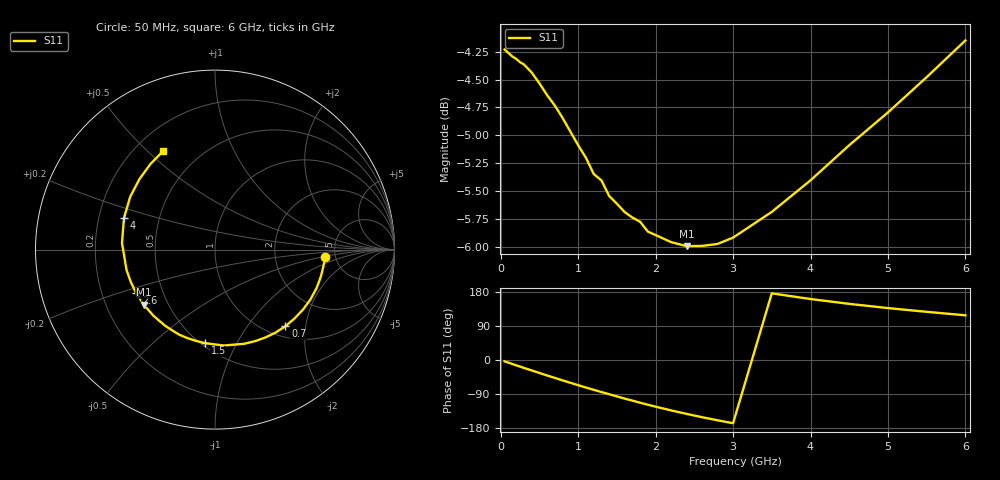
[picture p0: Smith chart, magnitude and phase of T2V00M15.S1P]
! SIEMENS Discrete & RF Semiconductors
! BAS70-04W
! Si Schottky Diode in SOT323
! IF = 0.15 mA
! S-Parameters:  November  1997
# GHz  S  MA  R  50
!  f  S11
! GHz  MAG  ANG
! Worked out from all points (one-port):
!   34 points, 50 MHz to 6 GHz, reference 50 ohm
!   lowest |S11| = -6.0 dB at 2.4 GHz (marker M1), VSWR 3.01, Z = 18.3 - j15 ohm
!   |S11| at or under -10 dB: nowhere
!   S11 on the Smith chart (normalised r, x): 50 MHz: 4.12, -0.51; 700 MHz: 1.20, -1.55; 1.5 GHz: 0.52, -0.75; 2.6 GHz: 0.35, -0.23; 4 GHz: 0.31, +0.15; 6 GHz: 0.31, +0.56
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0.05  0.6144 -3.6
0.15  0.61 -10.6
0.2  0.6085 -14.2
0.25  0.6064 -17.4
0.4  0.5999 -27.6
0.5  0.5933 -34.3
0.6  0.586 -41.0
0.7  0.5797 -47.4
0.8  0.5724 -53.9
0.9  0.5644 -60.2
1  0.5566 -66.5
1.1  0.5494 -72.7
1.3  0.5367 -84.6
1.5  0.5239 -96.1
1.6  0.5194 -101.8
1.8  0.5142 -112.8
2  0.5072 -123.2
2.2  0.5036 -133.0
2.4  0.5015 -142.2
2.6  0.5016 -151.0
2.8  0.5026 -159.1
3  0.5059 -166.9
3.5  0.5195 175.9
4  0.5368 160.9
4.5  0.5566 148.1
5  0.5757 137.0
5.5  0.5971 127.1
6  0.6202 117.9
